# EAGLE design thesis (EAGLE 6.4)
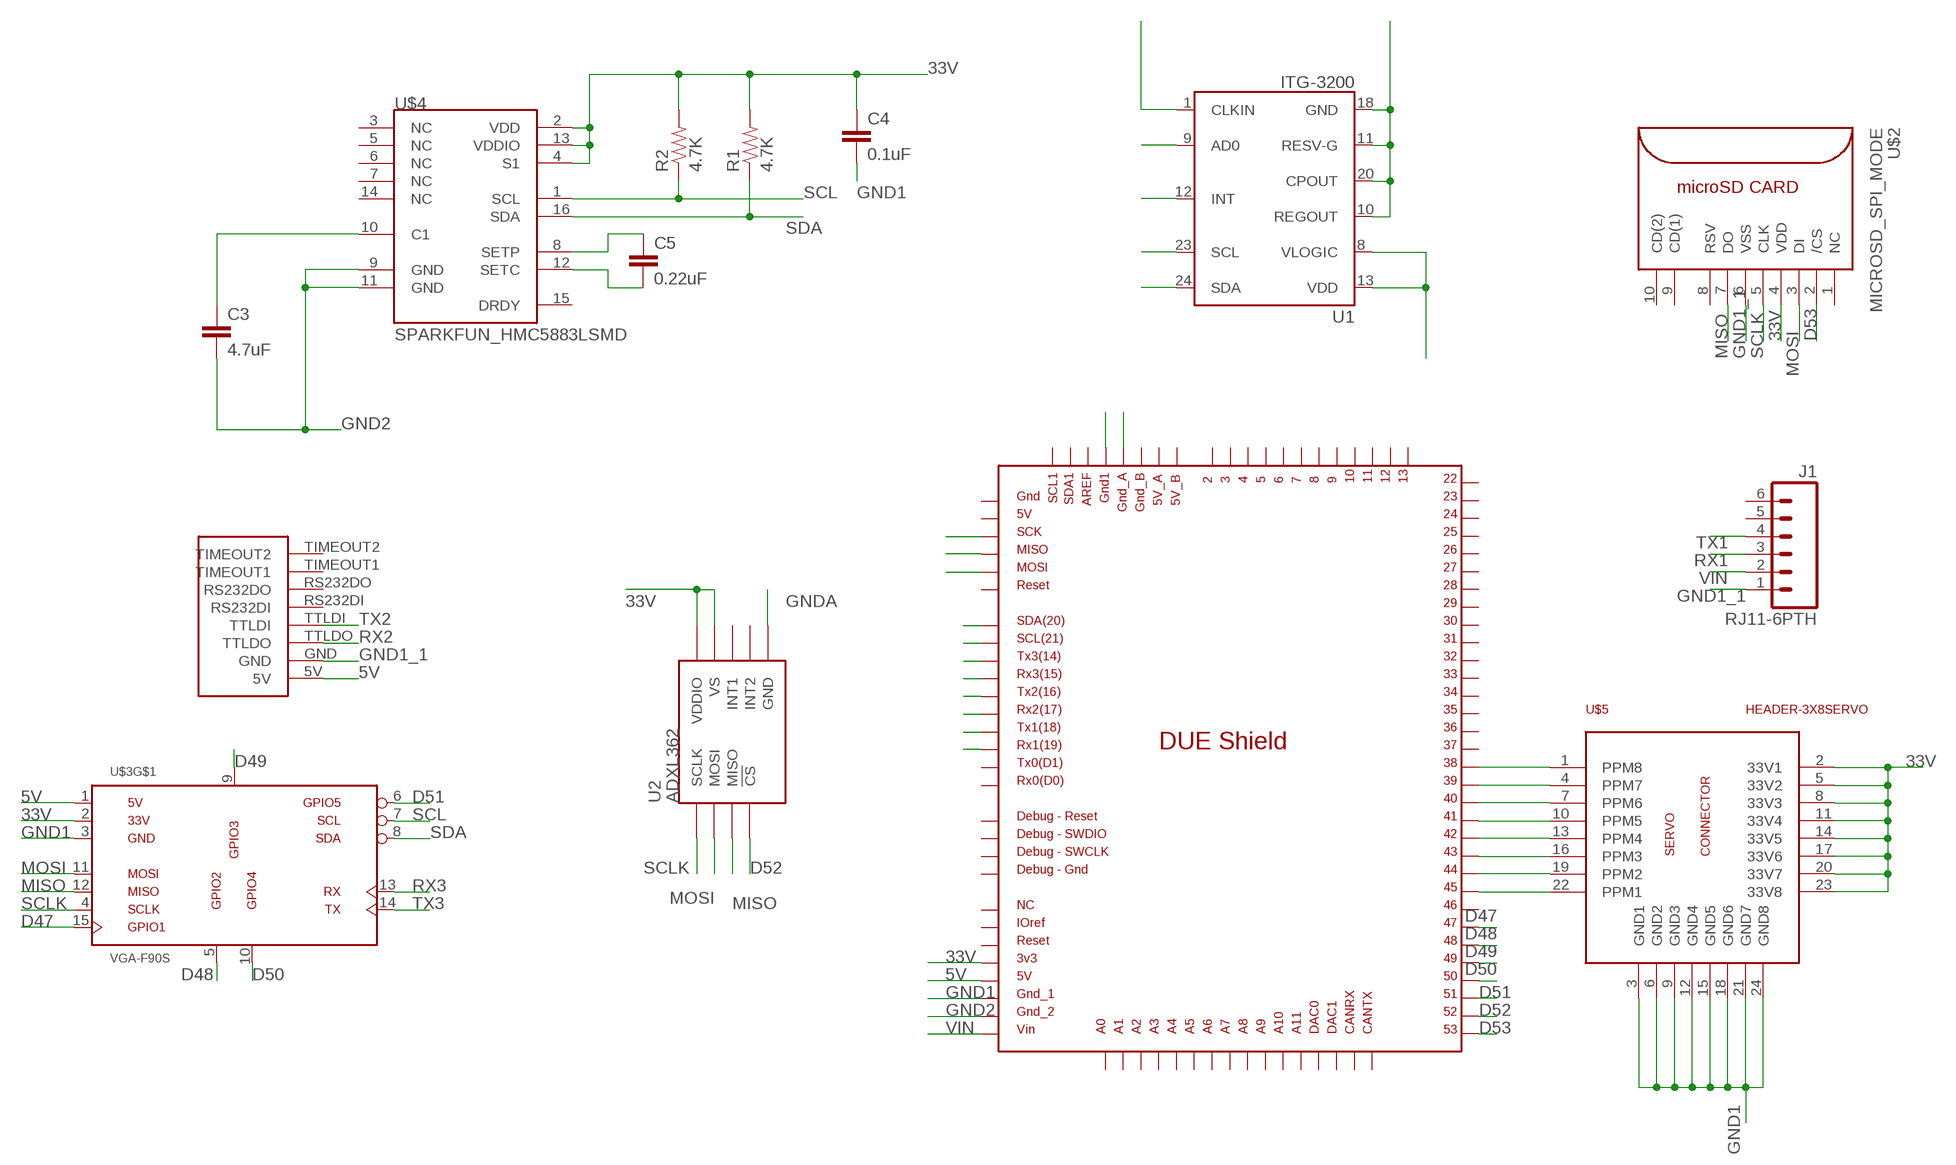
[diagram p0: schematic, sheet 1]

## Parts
C3  4.7uF  SPARKFUN_CAP0402-CAP  [SPARKFUN_0402-CAP]
C4  0.1uF  SPARKFUN_CAP0402-CAP  [SPARKFUN_0402-CAP]
C5  0.22uF  SPARKFUN_CAP0402-CAP  [SPARKFUN_0402-CAP]
J1  RJ11-6PTH  [RJ11-6]
R1  4.7K  SPARKFUN_RESISTOR0402-RES  [SPARKFUN_0402-RES]
R2  4.7K  SPARKFUN_RESISTOR0402-RES  [SPARKFUN_0402-RES]
U1  ITG-3200  [QFN-24]
U2  ADXL362  [ADXL362]
U$1  DUE(NORMAL)  [DUE(NORMAL)]
U$2  MICROSD_SPI_MODE  [MICRO_SD_CONNECTOR]
U$3  VGA-F90S  [DB-15-F90+SHIELD-SMALL_PADS]
U$4  SPARKFUN_HMC5883LSMD  [SPARKFUN_16LPCC]
U$5  HEADER-3X8SERVO  [3X8RA]
U$6  UBLOXLEA6TBOB  [UBLOXLEA6TBOB]

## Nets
5V: U$1.5V U$3.1(VGA-R) U$6.5V
33V: C4.1 R1.2 R2.2 U1.8(VLOGIC) U1.9(AD0) U1.13(VDD) U2.P$1(VDDIO) U2.P$14(VS) U$1.3V3 U$2.4(VDD) U$3.2(VGA-G) U$4.2(VDD) U$4.4(S1) U$4.13(VDDIO) U$5.2(33V1) U$5.5(33V2) U$5.8(33V3) U$5.11(33V4) U$5.14(33V5) U$5.17(33V6) U$5.20(33V7) U$5.23(33V8)
D47: U$1.47 U$3.15(ID3/SCL)
D48: U$1.48 U$3.5(GND)
D49: U$1.49 U$3.9(+5V)
D50: U$1.50 U$3.10(GND)
D51: U$1.51 U$3.6(VGA-R-)
D52: U2.P$8(!CS) U$1.52
D53: U$1.53 U$2.2(/CS)
GND1: C4.2 U$1.GND_1 U$3.3(VGA-B) U$5.3(GND1) U$5.6(GND2) U$5.9(GND3) U$5.12(GND4) U$5.15(GND5) U$5.18(GND6) U$5.21(GND7) U$5.24(GND8)
GND1_1: J1.1 U$1.GND1 U$2.6(VSS) U$6.GND
GND2: C3.2 U$1.GND_2 U$4.9(GND) U$4.11(GND)
GNDA: U1.1(CLKIN) U1.10(REGOUT) U1.11(RESV-G) U1.12(INT) U1.18(GND) U1.20(CPOUT) U2.P$12(GND) U2.P$13(GND) U2.P$16(GND) U$1.GND_A
MISO: U2.P$7(MISO) U$1.MISO_ICSP U$2.7(DO) U$3.12(ID1/SDA)
MOSI: U2.P$6(MOSI) U$1.MOSI_ICSP U$2.3(DI) U$3.11(ID0/RES)
N$1: U$1.38 U$5.1(PPM8)
N$2: U$1.39 U$5.4(PPM7)
N$3: U$1.40 U$5.7(PPM6)
N$4: U$1.41 U$5.10(PPM5)
N$5: C5.1 U$4.8(SETP)
N$6: U$1.42 U$5.13(PPM4)
N$7: C5.2 U$4.12(SETC)
N$8: U$1.43 U$5.16(PPM3)
N$9: U$1.44 U$5.19(PPM2)
N$10: U$1.45 U$5.22(PPM1)
N$12: C3.1 U$4.10(C1)
RX1: J1.3 U$1.RX1
RX2: U$1.RX2 U$6.TTLDO
RX3: U$1.RX3 U$3.13(VGA-HSYNC)
SCL: R2.1 U1.23(SCL) U$1.SCL U$3.7(VGA-G-) U$4.1(SCL)
SCLK: U2.P$4(SCLK) U$1.SCK_ICSP U$2.5(CLK) U$3.4(ID2/RES)
SDA: R1.1 U1.24(SDA) U$1.SDA U$3.8(VGA-B-) U$4.16(SDA)
TX1: J1.4 U$1.TX1
TX2: U$1.TX2 U$6.TTLDI
TX3: U$1.TX3 U$3.14(VGA-VSYNC)
VIN: J1.2 U$1.VIN
Unconnected: J1.5 J1.6 U2.P$9(INT2) U2.P$11(INT1) U$1.2 U$1.3 U$1.4 U$1.5 U$1.5V_A U$1.5V_B U$1.5V_ICSP U$1.6 U$1.7 U$1.8 U$1.9 U$1.10 U$1.11 U$1.12 U$1.13 U$1.22 U$1.23 U$1.24 U$1.25 U$1.26 U$1.27 U$1.28 U$1.29 U$1.30 U$1.31 U$1.32 U$1.33 U$1.34 U$1.35 U$1.36 U$1.37 U$1.46 U$1.A0 U$1.A1 U$1.A2 U$1.A3 U$1.A4 U$1.A5 U$1.A6 U$1.A7 U$1.A8 U$1.A9 U$1.A10 U$1.A11 U$1.AREF U$1.CANRX U$1.CANTX U$1.DAC0 U$1.DAC1 U$1.GND_B U$1.GND_DEBUG U$1.GND_ICSP U$1.IOREF U$1.NC U$1.RESET U$1.RESET_DEBUG U$1.RESET_ICSP U$1.RX0 U$1.SCL1 U$1.SDA1 U$1.SWCLK_DEBUG U$1.SWDIO_DEBUG U$1.TX0 U$2.1(NC) U$2.8(RSV) U$2.9(CD(1)) U$2.10(CD(2)) U$3.SHIELD@1(SHIELD) U$3.SHIELD@2(SHIELD) U$4.3(NC) U$4.5(NC) U$4.6(NC) U$4.7(NC) U$4.14(NC) U$4.15(DRDY) U$6.RS232DI U$6.RS232DO U$6.TIMEOUT1 U$6.TIMEOUT2

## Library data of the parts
C3-C5 = HMC5883L_Breakout-v11:SPARKFUN_CAP: Capacitor
J1 = SparkFun-Connectors:RJ11-6: RJ11 Jack Simple 6 pin RJ11 jack. Commonly found on CAT3 devices and Microchip programmers. SKU: PRT-00132
R1 R2 = HMC5883L_Breakout-v11:SPARKFUN_RESISTOR: Resistor
U1 = SparkFun:ITG-3200: ITG-3200 3-axis gyro, digital output, qfn24 package
U2 = SparkFun-Sensors:ADXL362: Micropower 3-axis accelerometer 2/4/8g digital output (SPI) IC-11297; PROD_ID: IC-11297
U$1 = DUElib130425:DUE(NORMAL)
U$2 = con-molex-microsd:MICROSD_SPI_MODE: MOLEX - 49225-0821 - CONNECTEUR MICRO SD PUSH/PUSH REV Fabricant: MOLEX Code commande Farnell: 1366700 Référence fabricant: 49225-0821
U$3 = VideoConnectors:VGA-*
U$4 = HMC5883L_Breakout-v11:SPARKFUN_HMC5883L: 3 Axis Digital Compass IC
U$5 = pixhawk2:HEADER-3X8
U$6 = csgshop:UBLOXLEA6TBOB

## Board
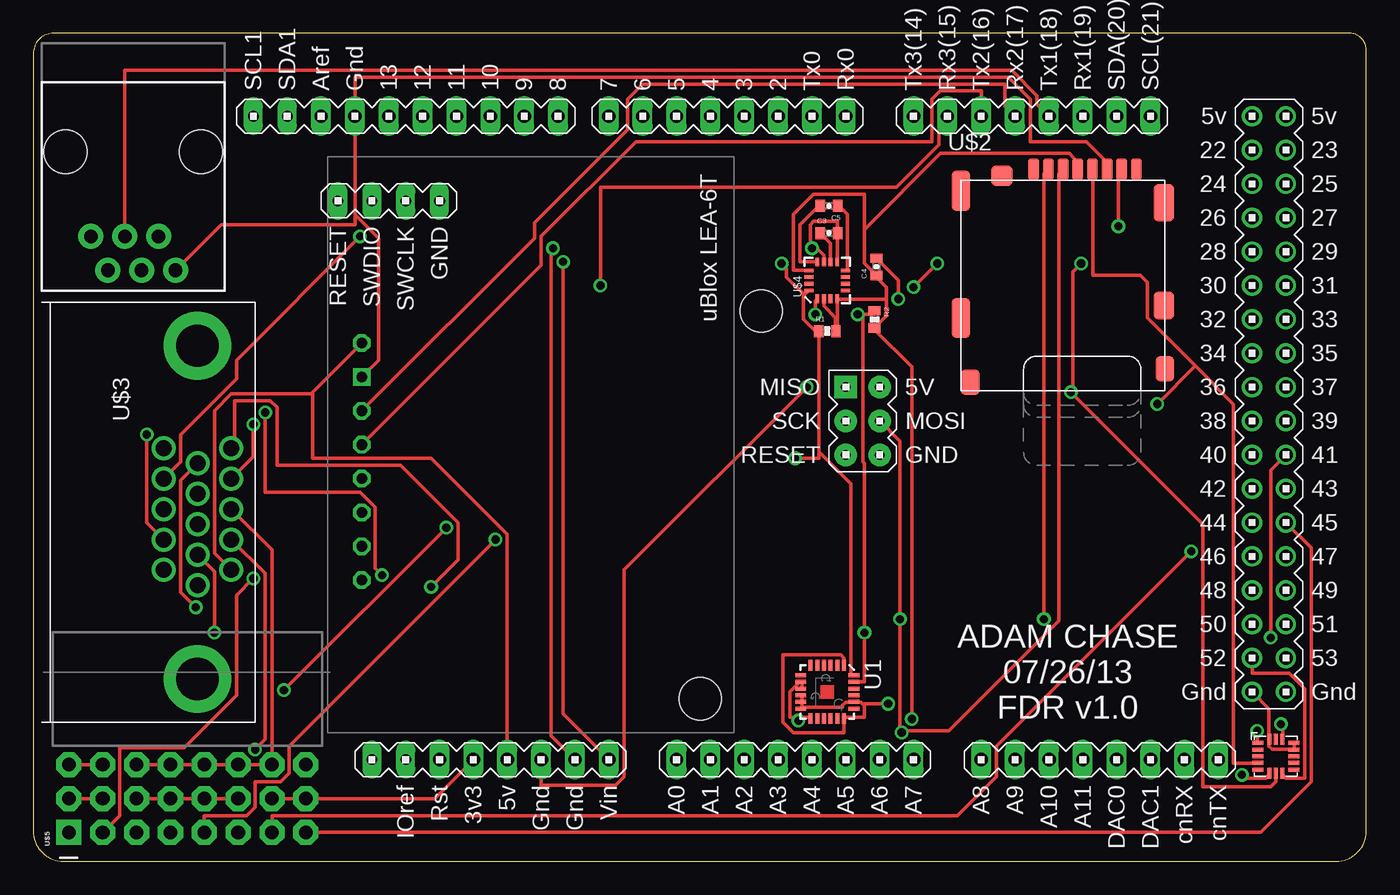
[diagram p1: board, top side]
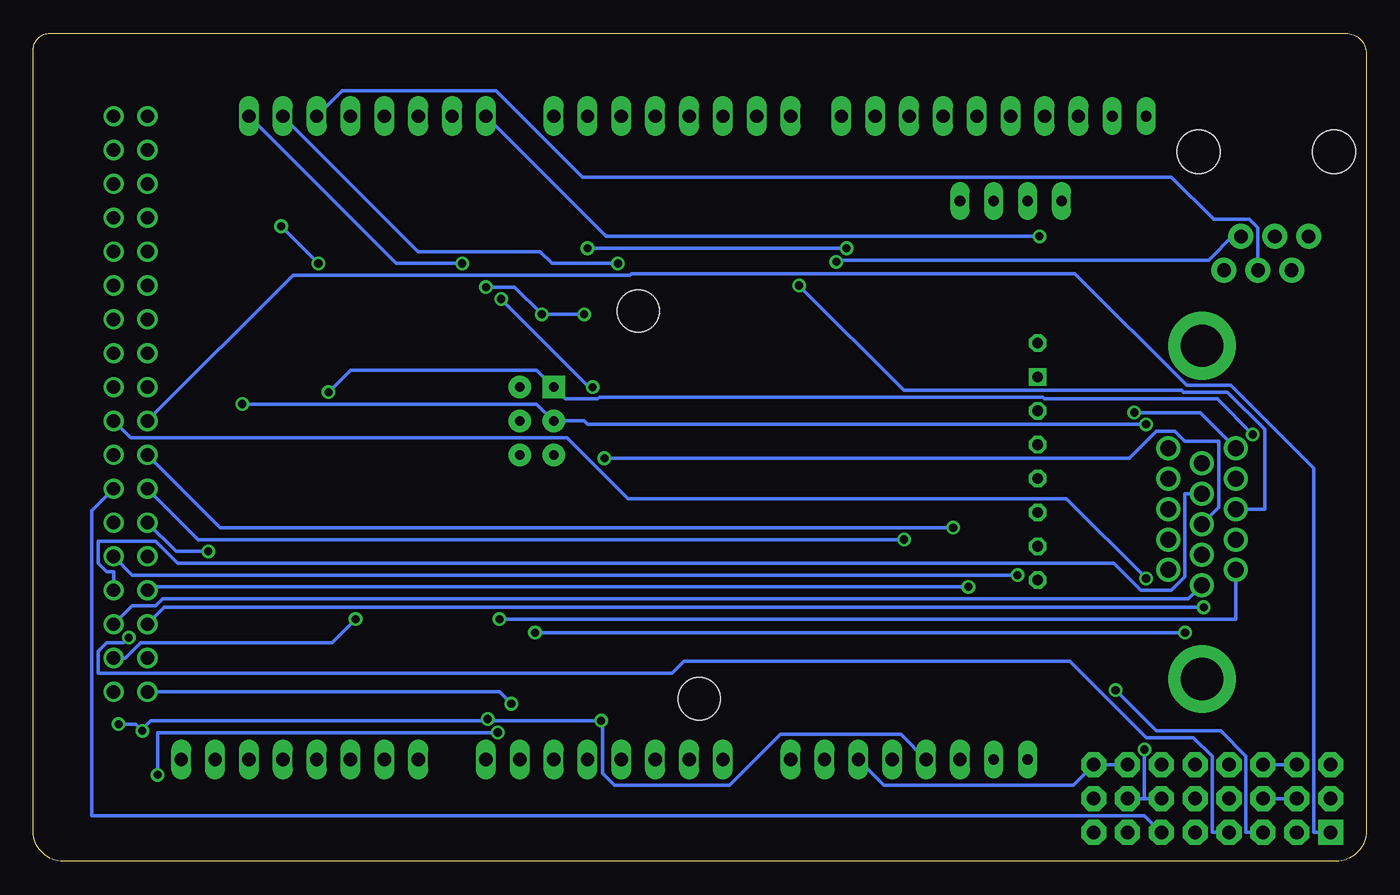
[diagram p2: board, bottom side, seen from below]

Size 100 x 62.09 mm. Coordinates in mm from the lower left corner, seen from the top.
Outline: 100,2.25 100,60.87 arc90 98.78,62.09 1.52,62.09 arc90 0,60.57 0,2.26 arc90 2.26,0 97.75,0 arc90 100,2.25
Copper layers (1*16): Top 0.035mm / dielectric 1.5mm / Bottom 0.035mm
Design rules "default": minimum track width 10mil, minimum drill 24mil, track to track 8mil, track to pad 8mil, pad to pad 8mil, via to via 8mil, smd to smd 8mil, copper to edge 40mil, drill to drill 8mil, minimum pad ring 10mil, minimum via ring 8mil, stop-mask expansion 4mil, vias tented up to drill 0mil, thermal gap 10mil
Holes 3.17 mm at 54.61,41.27

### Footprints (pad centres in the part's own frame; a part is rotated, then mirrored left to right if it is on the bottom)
SPARKFUN_0402-CAP = smd 0.7 x 0.9: 1 -0.65,0; 2 0.65,0
RJ11-6 = drill 1.016 pad 1.88: 1 1.905,8.89; 2 3.175,6.35; 3 4.445,8.89; 4 5.715,6.35; 5 6.985,8.89; 6 8.255,6.35 | hole 3.251: 0,0; 10.16,0
SPARKFUN_0402-RES = smd 0.7 x 0.9: 1 -0.65,0; 2 0.65,0
QFN-24 = smd 0.8 x 0.3: 1 -2,1.25; 2 -2,0.75; 3 -2,0.25; 4 -2,-0.25; 5 -2,-0.75; 6 -2,-1.25; 13 2,-1.25; 14 2,-0.75; 15 2,-0.25; 16 2,0.25; 17 2,0.75; 18 2,1.25 | smd 0.3 x 0.8: 7 -1.25,-2; 8 -0.75,-2; 9 -0.25,-2; 10 0.25,-2; 11 0.75,-2; 12 1.25,-2; 19 1.25,2; 20 0.75,2; 21 0.25,2; 22 -0.25,2; 23 -0.75,2; 24 -1.25,2
ADXL362 = smd 0.8 x 0.3: P$1 -1.35,1; P$2 -1.35,0.5; P$3 -1.35,0; P$4 -1.35,-0.5; P$5 -1.35,-1; P$9 1.35,-1; P$10 1.35,-0.5; P$11 1.35,0; P$12 1.35,0.5; P$13 1.35,1 | smd 0.3 x 0.8: P$6 -0.5,-1.275; P$7 0,-1.275; P$8 0.5,-1.275; P$14 0.5,1.275; P$15 0,1.275; P$16 -0.5,1.275
DUE(NORMAL) = drill 1 long: 2 -16.51,30.48; 3 -19.05,30.48; 3V3 -39.37,-17.78; 4 -21.59,30.48; 5 -24.13,30.48; 5V -36.83,-17.78; 6 -26.67,30.48; 7 -29.21,30.48; 8 -33.02,30.48; 9 -35.56,30.48; 10 -38.1,30.48; 11 -40.64,30.48; 12 -43.18,30.48; 13 -45.72,30.48; A0 -24.13,-17.78; A1 -21.59,-17.78; A2 -19.05,-17.78; A3 -16.51,-17.78; A4 -13.97,-17.78; A5 -11.43,-17.78; A6 -8.89,-17.78; A7 -6.35,-17.78; A8 -1.27,-17.78; A9 1.27,-17.78; A10 3.81,-17.78; A11 6.35,-17.78; AREF -50.8,30.48; AREF1 -50.8,30.48; CANRX 13.97,-17.78; CANTX 16.51,-17.78; DAC0 8.89,-17.78; DAC1 11.43,-17.78; GND1 -48.26,30.48; GND_1 -34.29,-17.78; GND_2 -31.75,-17.78; RESET -41.91,-17.78; RX0 -11.43,30.48; RX1 6.35,30.48; RX2 1.27,30.48; RX3 -3.81,30.48; SCL 11.43,30.48; SDA 8.89,30.48; TX0 -13.97,30.48; TX1 3.81,30.48; TX2 -1.27,30.48; TX3 -6.35,30.48; VIN -29.21,-17.78 | drill 1: 5V_A 19.05,30.48; 5V_B 21.59,30.48; 22 19.05,27.94; 23 21.59,27.94; 24 19.05,25.4; 25 21.59,25.4; 26 19.05,22.86; 27 21.59,22.86; 28 19.05,20.32; 29 21.59,20.32; 30 19.05,17.78; 31 21.59,17.78; 32 19.05,15.24; 33 21.59,15.24; 34 19.05,12.7; 35 21.59,12.7; 36 19.05,10.16; 37 21.59,10.16; 38 19.05,7.62; 39 21.59,7.62; 40 19.05,5.08; 41 21.59,5.08; 42 19.05,2.54; 43 21.59,2.54; 44 19.05,0; 45 21.59,0; 46 19.05,-2.54; 47 21.59,-2.54; 48 19.05,-5.08; 49 21.59,-5.08; 50 19.05,-7.62; 51 21.59,-7.62; 52 19.05,-10.16; 53 21.59,-10.16; GND_A 19.05,-12.7; GND_B 21.59,-12.7 | drill 0.7 pad 1.676: 5V_ICSP -8.89,5.08; GND_ICSP -8.89,10.16; MOSI_ICSP -8.89,7.62; RESET_ICSP -11.43,5.08; SCK_ICSP -11.43,7.62 | drill 0.8 pad 1.422 long: GND_DEBUG -41.91,24.13; IOREF -44.45,-17.78; NC -46.99,-17.78; RESET_DEBUG -49.53,24.13; SCL1 -55.88,30.48; SDA1 -53.34,30.48; SWCLK_DEBUG -44.45,24.13; SWDIO_DEBUG -46.99,24.13 | drill 0.7 pad 1.676 square: MISO_ICSP -11.43,10.16
MICRO_SD_CONNECTOR = smd 0.8 x 1.6: 1 -2.03,8.2; 2 -0.93,8.2; 3 0.17,8.2; 4 1.27,8.2; 5 2.37,8.2; 6 3.47,8.2; 7 4.57,8.2; 8 5.67,8.2 | smd 1.55 x 2.8: 9 7.735,5.7 | smd 1.55 x 2.1: 10 7.735,-2 | smd 1.4 x 1.9: 11 7.81,-6.75; 12 -6.79,-7.75 | smd 1.4 x 3: 13 -7.49,-2.95; 14 -7.49,6.6 | smd 1.6 x 1.55: 15 -4.43,7.725
DB-15-F90+SHIELD-SMALL_PADS = drill 1.2 pad 1.524: 1 4.318,14.224; 2 2.032,14.224; 3 -0.254,14.224; 4 -2.54,14.224; 5 -4.826,14.224; 6 5.461,11.684; 7 3.175,11.684; 8 0.889,11.684; 9 -1.397,11.684; 10 -3.683,11.684; 11 4.318,9.144; 12 2.032,9.144; 13 -0.254,9.144; 14 -2.54,9.144; 15 -4.826,9.144 | drill 3.175 pad 5.08: SHIELD@1 -12.497,11.684; SHIELD@2 12.497,11.684
SPARKFUN_16LPCC = smd 0.65 x 0.28: 1 -1.37,0.75; 2 -1.37,0.25; 3 -1.37,-0.25; 4 -1.37,-0.75; 9 1.37,-0.75; 10 1.37,-0.25; 11 1.37,0.25; 12 1.37,0.75 | smd 0.28 x 0.65: 5 -0.75,-1.37; 6 -0.25,-1.37; 7 0.25,-1.37; 8 0.75,-1.37; 13 0.75,1.37; 14 0.25,1.37; 15 -0.25,1.37; 16 -0.75,1.37
3X8RA = drill 1.016 pad 1.88 square: 1 -1.27,8.89 | drill 1.016 pad 1.88 octagon: 2 1.27,8.89; 3 3.81,8.89; 4 -1.27,6.35; 5 1.27,6.35; 6 3.81,6.35; 7 -1.27,3.81; 8 1.27,3.81; 9 3.81,3.81; 10 -1.27,1.27; 11 1.27,1.27; 12 3.81,1.27; 13 -1.27,-1.27; 14 1.27,-1.27; 15 3.81,-1.27; 16 -1.27,-3.81; 17 1.27,-3.81; 18 3.81,-3.81; 19 -1.27,-6.35; 20 1.27,-6.35; 21 3.81,-6.35; 22 -1.27,-8.89; 23 1.27,-8.89; 24 3.81,-8.89
UBLOXLEA6TBOB = drill 0.8 octagon: 5V 13.97,2.54; RS232DI 24.13,2.54; RS232DO 26.67,2.54; TIMEOUT1 29.21,2.54; TIMEOUT2 31.75,2.54; TTLDI 21.59,2.54; TTLDO 19.05,2.54 | drill 0.8 square: GND 16.51,2.54 | hole 3.175: 40.64,27.94

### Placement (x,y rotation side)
C3  59.69,47.12 0 top
C4  63.25,44.58 90 top
C5  59.69,49.15 180 top
J1  12.57,53.21 180 top
R1  59.56,39.75 0 top
R2  63.12,40.64 270 top
U1  59.56,12.7 270 top
U2  93.22,7.87 0 top
U$1  72.39,25.4 0 top
U$2  77.09,43.69 0 top
U$3  0.64,26.16 270 top
U$4  59.56,43.56 90 top
U$5  11.56,3.43 90 top
U$6  22.1,52.83 270 top

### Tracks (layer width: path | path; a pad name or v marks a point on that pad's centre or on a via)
5V
  Top 0.254: 20.89,35.12 20.83,35.05 14.86,35.05 13.59,33.78 13.59,23.11 U$3.1 | 20.89,35.12 U$6.5V | U$1.5V 35.56,24.51 29.84,30.23 20.95,30.23 20.95,35.05 20.89,35.12
33V  (via drill 0.61)
  Top 0.254: U$1.3V3 30.1,4.7 U$5.23 U$5.20 | U$5.5 U$5.2 | U$5.8 U$5.11 U$5.14 U$5.17 | U$3.2 17.4,21.59 17.4,9.14 v16.64,8.38 | U$4.2 59.31,42.16 59.31,41.66 60.2,40.77 60.2,39.75 R1.2 60.33,39.75 60.33,42.16 U$4.4 60.45,42.16 64.01,42.16 | 62.36,47.37 62.36,44.83 63.25,43.94 C4.1 63.25,43.81 64.01,43.05 64.01,42.16 | 62.36,47.37 62.36,50.04 58.55,50.04 57.02,48.51 57.02,44.32 58.17,44.32 U$4.13 | 64.01,42.16 64.01,40.89 63.12,40.01 R2.2 63.12,39.88 65.91,37.08 v65.91,10.67 | 62.36,47.37 68.07,53.09 77.72,53.09 78.11,52.7 78.11,52.2 78.36,51.94 U$2.4 | v91.82,9.78 91.82,8.89 U2.P$1 | v93.6,10.29 93.73,10.16 93.73,9.27 U2.P$14 | U1.9 57.66,12.95 57.66,13.34 U1.8 57.53,13.46 56.77,12.7 56.77,10.79 57.4,10.79 | 57.4,10.79 58.29,10.79 U1.13 | 57.4,10.79 v57.4,10.54
  Bottom 0.254: U$5.8 U$5.5 | 16.64,4.7 v16.64,8.38 | U$5.17 16.64,4.7 | 16.64,4.7 U$5.20 | v93.6,10.29 92.33,10.29 v91.82,9.78 91.82,9.91 91.19,10.54 65.91,10.54 | 65.91,10.54 v57.4,10.54 57.28,10.54 57.28,6.6 56.39,5.71 47.75,5.71 43.94,9.53 34.92,9.53 U$1.3V3 | 65.91,10.54 v65.91,10.67
D47  (via drill 0.61)
  Top 0.254: v26.16,21.46 25.65,21.97 25.65,26.54 24.51,27.69 17.4,27.69 v17.4,33.66
  Bottom 0.254: U$1.47 92.58,21.46 v26.16,21.46 | v17.4,33.66 12.45,33.66 U$3.15
D48  (via drill 0.61)
  Top 0.254: v29.84,20.57 31.88,22.61 31.88,25.4 27.56,29.72 18.29,29.72 18.29,34.04 17.78,34.54 15.11,34.54 15.11,31.24 U$3.5
  Bottom 0.254: U$1.48 91.19,20.57 v29.84,20.57
D49
  Bottom 0.254: U$1.49 93.98,21.72 94.49,21.72 95.12,22.35 95.12,24 90.81,24 89.15,22.35 18.92,22.35 16.89,20.32 14.61,20.32 13.59,21.34 13.59,27.56 U$3.9
D50  (via drill 0.61)
  Top 0.254: v12.19,19.05 11.05,20.19 11.05,28.57 U$3.10
  Bottom 0.254: U$1.50 90.17,19.05 v12.19,19.05
D51
  Bottom 0.254: U$1.51 92.58,19.18 90.81,19.18 90.3,19.68 13.34,19.68 U$3.6
D52
  Top 0.254: U$1.52 91.44,14.1 94.23,14.1 95.38,12.95 95.38,6.22 93.98,6.22 93.73,6.48 U2.P$8
D53  (via drill 0.61)
  Top 0.254: v75.82,18.16 75.82,51.56 76.07,51.82 U$2.2
  Bottom 0.254: v75.82,18.16 77.6,16.38 91.95,16.38 93.09,15.24 U$1.53
GND1  (via drill 0.61)
  Top 0.254: U$5.6 U$5.3 | U$5.9 U$5.12 U$5.15 U$5.18 U$5.21 17.91,23.37 U$3.3 | v64.9,42.16 64.9,43.56 63.25,45.21 C4.2 | v58.04,35.56 44.32,21.84 44.32,6.35 43.69,5.71 38.1,5.71 U$1.GND_1
  Bottom 0.254: U$5.9 U$5.6 | U$5.21 U$5.24 21.97,5.71 36.2,5.71 U$1.GND_1 | v64.9,42.16 58.29,35.56 v58.04,35.56
GND1_1
  Top 0.254: U$2.6 80.52,51.94 80.26,52.2 80.26,52.7 78.99,53.98 74.8,53.98 74.8,57.15 73.15,58.8 24.13,58.8 U$1.GND1 24.13,48.51 24.19,48.45 | U$6.GND 25.91,37.59 25.91,46.74 24.19,48.45 | J1.1 14.1,47.75 24.13,47.75 24.13,48.39 24.19,48.45
GND2  (via drill 0.61)
  Top 0.254: 58.61,46.16 58.29,46.48 58.29,47.75 58.55,48.01 60.33,48.01 60.33,47.12 | 58.61,46.16 59.31,45.47 59.31,44.96 U$4.11 | 60.33,47.12 60.33,44.96 U$4.9 | 60.33,47.12 C3.2 | v58.42,45.97 58.61,46.16 | v38.99,45.97 38.86,45.85 38.86,9.4 U$1.GND_2
  Bottom 0.254: v38.99,45.97 v58.42,45.97
GNDA  (via drill 0.61)
  Top 0.254: U1.10 57.66,12.45 57.66,12.06 U1.11 57.66,11.94 57.66,11.56 U1.12 57.78,11.56 60.71,11.56 60.71,11.68 60.96,11.94 61.47,11.94 U1.20 61.59,11.94 62.1,11.94 62.29,11.75 | 62.29,11.75 62.36,11.68 62.36,10.79 60.83,10.79 U1.18 60.83,10.67 60.83,9.65 57.02,9.65 56.26,10.41 56.26,15.49 60.58,15.49 60.83,15.24 60.83,14.73 U1.1 | U2.P$13 94.61,8.76 94.61,8.38 U2.P$12 94.49,8.38 92.96,8.38 92.71,8.64 U2.P$16 92.71,9.27 92.71,11.43 U$1.GND_A | v64.14,11.81 62.36,11.81 62.29,11.75
  Bottom 0.254: v64.14,11.81 65.02,12.7 U$1.GND_A
MISO  (via drill 0.61)
  Top 0.254: U2.P$7 93.22,5.97 92.84,5.59 87.76,5.59 87.76,25.27 v77.85,35.18 77.98,35.18 77.98,44.2 v78.61,44.83 | v81.41,47.62 81.41,51.69 81.53,51.82 U$2.7 | U$3.12 8.51,25.4 v8.51,32
  Bottom 0.254: v77.85,35.18 76.2,36.83 62.23,36.83 U$1.MISO_ICSP 60.07,34.67 57.66,34.67 57.53,34.8 24.26,34.8 24.13,34.67 11.18,34.67 v8.51,32 | v78.61,44.83 v81.41,47.62
MOSI  (via drill 0.61)
  Top 0.254: v90.68,6.48 90.68,6.22 92.46,6.22 92.71,6.48 U2.P$6 | U$1.MOSI_ICSP 65.02,31.5 v65.02,18.16 65.02,9.78 v65.15,9.65 65.15,9.78 68.71,9.78 76.96,18.03 76.96,51.56 77.22,51.82 U$2.3
  Bottom 0.254: v90.68,6.48 90.68,9.65 v65.15,9.65 | U$3.11 9.78,18.16 v65.02,18.16
N$1
  Bottom 0.254: U$1.38 80.52,43.94 55.24,43.94 55.12,44.07 21.84,44.07 13.46,35.69 10.16,35.69 3.94,29.46 3.94,2.16 U$5.1
N$2  (via drill 0.61)
  Top 0.254: v16.51,21.21 15.24,19.94 15.24,12.45 11.3,8.51 6.48,8.51 6.48,3.43 U$5.4
  Bottom 0.254: U$1.39 92.71,31.75 59.94,31.75 55.37,27.18 22.48,27.18 v16.51,21.21
N$3  (via drill 0.61)
  Top 0.254: v18.8,12.83 v30.99,25.02
  Bottom 0.254: U$1.40 85.98,25.02 v30.99,25.02 | v18.8,12.83 15.75,9.78 10.92,9.78 9.02,7.87 9.02,2.16 U$5.7
N$4  (via drill 0.61)
  Top 0.254: U$1.41 92.84,29.34 v92.84,16.76
  Bottom 0.254: v92.84,16.76 93.22,16.38 94.49,16.38 95.12,15.75 95.12,14.1 52.07,14.1 51.18,14.99 22.23,14.99 16.51,9.27 12.95,9.27 11.56,7.87 11.56,2.16 U$5.10
N$5
  Top 0.254: U$4.8 60.96,44.32 61.09,44.45 61.09,48.51 60.45,49.15 C5.1
N$6  (via drill 0.61)
  Top 0.254: v34.67,24.13 19.18,8.64 19.18,6.6 18.54,5.97 16.64,5.97 16.64,4.06 16,3.43 12.83,3.43 U$5.13
  Bottom 0.254: U$1.42 87.63,24.13 v34.67,24.13
N$7
  Top 0.254: U$4.12 58.8,44.96 57.53,44.96 57.53,47.75 58.93,49.15 C5.2
N$8
  Bottom 0.254: U$1.43 95.63,26.29 95.63,3.43 16.64,3.43 U$5.16
N$9  (via drill 0.61)
  Top 0.254: v86.87,23.24 72.26,8.64 72.26,6.35 69.34,3.43 17.91,3.43 U$5.19
  Bottom 0.254: U$1.44 89.28,23.24 v86.87,23.24
N$10
  Top 0.254: U$1.45 95.89,23.5 95.89,5.97 92.08,2.16 U$5.22
N$12
  Top 0.254: U$4.10 59.82,44.96 59.82,46.35 59.05,47.12 C3.1
RX1
  Bottom 0.254: U$1.RX1 76.83,57.78 65.28,57.78 58.8,51.31 14.61,51.31 11.43,48.13 8.76,48.13 8.13,47.5 J1.3
RX2
  Top 0.254: U$6.TTLDO 37.59,46.74 37.59,47.88 44.58,54.86 44.58,57.15 45.72,58.29 72.9,58.29 72.9,56.64 U$1.RX2
RX3  (via drill 0.61)
  Top 0.254: U$1.RX3 67.94,55.24 67.94,53.72 64.77,50.55 42.55,50.55 v42.55,43.18
  Bottom 0.254: v42.55,43.18 34.67,35.31 13.84,35.31 13.72,35.18 10.41,35.18 7.62,32.38 7.62,26.42 U$3.13
SCL  (via drill 0.61)
  Top 0.254: v58.67,41.02 58.67,42.04 58.8,42.16 U$4.1 | 62.23,41.02 63.12,41.02 R2.1 | 62.23,41.02 62.23,29.97 62.36,29.84 v62.36,17.14 62.36,13.46 61.59,13.46 U1.23 | 62.23,41.02 v61.85,41.02 | v66.04,43.05 v67.82,44.83 | U$3.7 13.59,21.72 v13.59,17.14
  Bottom 0.254: v58.67,41.02 v61.85,41.02 63.88,43.05 v66.04,43.05 | U$1.SCL 72.77,44.83 v67.82,44.83 | v62.36,17.14 v13.59,17.14
SCLK  (via drill 0.61)
  Top 0.254: 87.19,37.15 83.57,40.77 83.57,43.43 83.06,43.94 79.5,43.94 79.5,51.82 U$2.5 | 87.19,37.15 90.04,34.29 90.04,7.37 91.82,7.37 U2.P$4 | 87.19,37.15 v84.33,34.29 | U$3.4 16.51,30.35 v16.51,32.77
  Bottom 0.254: v84.33,34.29 62.23,34.29 U$1.SCK_ICSP 58.67,33.02 58.42,32.77 v16.51,32.77
SDA  (via drill 0.61)
  Top 0.254: 57.85,42.48 57.78,42.42 57.78,40.64 58.67,39.75 R1.1 58.93,39.75 58.93,30.73 58.99,30.67 | 57.85,42.48 58.17,42.8 U$4.16 | 58.99,30.67 61.34,28.32 61.34,14.1 61.47,13.97 U1.24 | v56.13,44.83 56.52,44.45 56.52,43.81 57.85,42.48 | v57.15,30.23 58.93,30.23 58.93,30.61 58.99,30.67
  Bottom 0.254: U$1.SDA 71.12,45.72 61.98,45.72 61.09,44.83 v56.13,44.83 | U$3.8 11.05,26.54 11.05,31.5 13.59,31.5 14.35,32.26 15.75,32.26 17.78,30.23 v57.15,30.23
TX1
  Top 0.254: U$1.TX1 75.31,56.77 75.31,57.4 73.41,59.31 6.86,59.31 J1.4
TX2
  Top 0.254: U$6.TTLDI 38.1,44.7 38.1,46.86 45.21,53.98 67.44,53.98 67.44,57.15 68.07,57.78 71.12,57.78 U$1.TX2
TX3  (via drill 0.61)
  Top 0.254: v24.51,46.86 15.24,37.59 15.24,36.2 11.05,32 11.05,29.97 U$3.14
  Bottom 0.254: U$1.TX3 57.02,46.86 v24.51,46.86
VIN  (via drill 0.61)
  Top 0.254: U$1.VIN 39.75,11.05 v39.75,44.96
  Bottom 0.254: v39.75,44.96 39.62,45.09 11.81,45.09 10.03,46.86 J1.2

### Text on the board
tPlace: ADAM CHASE / 07/26/13 / FDR v1.0

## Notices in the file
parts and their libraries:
SparkFun-Sensors: Licensing: CC v3.0 Share-Alike You are welcome to use this library for commercial purposes.
